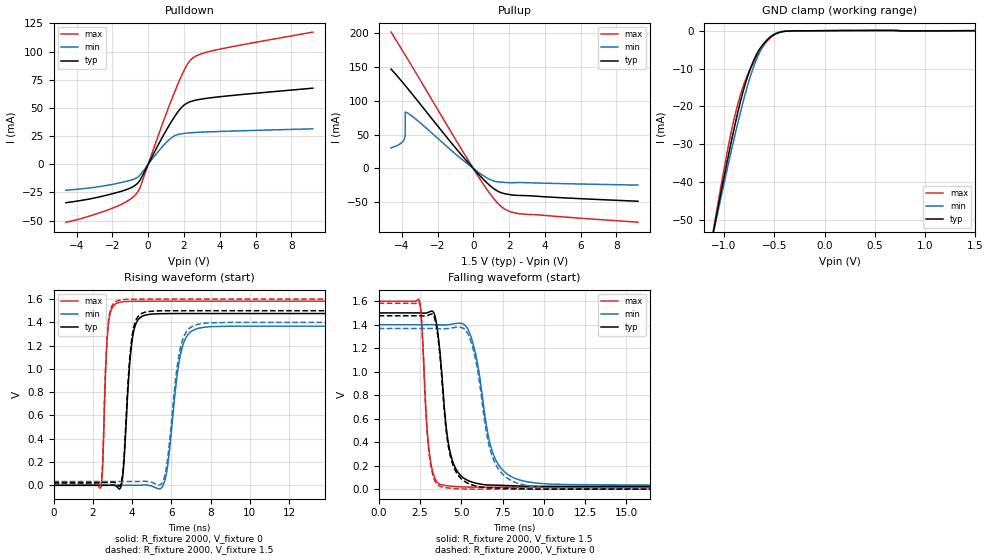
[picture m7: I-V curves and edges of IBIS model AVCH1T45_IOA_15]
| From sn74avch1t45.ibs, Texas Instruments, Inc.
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[Model]   AVCH1T45_IOA_15
Model_type  I/O
Vinl=0.49
Vinh=1.04
Enable   Active-Low
Vref =   0
Rref =   2000
Cref =   15p
Vmeas =   0.75
| variable   typ   min   max
C_comp   5.30pF   4.64pF   5.89pF
| C_pullup   5.23pF   3.72pF   7.65pF
| C_pulldown   4.92pF   4.34pF   5.58pF
| C_tri-state   5.30pF   4.64pF   5.89pF
[Temperature Range]   40   100   -40
| Ambient temperature   25   85   -40
[Voltage range]   1.5   1.4   1.6
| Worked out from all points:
|   slope of the pulldown table from 0 to 0.225 V, typ, clamps not added: 32.1 ohm
|   slope of the pullup table from 0 to 0.225 V, typ, clamps not added: 33.9 ohm
|   GND clamp passes 1 mA (typ) near -0.50 V on its own axis
|   rising waveform, R_fixture 2000, V_fixture 0: 20-80 % time 334ps typ, 544ps min, 203ps max; typ from 0 V to 1.48 V
|   falling waveform, R_fixture 2000, V_fixture 1.5: 20-80 % time 639ps typ, 1.02ns min, 391ps max; typ from 1.5 V to 0.023 V
|   rising waveform, R_fixture 2000, V_fixture 1.5: 20-80 % time 330ps typ, 532ps min, 202ps max; typ from 0.023 V to 1.5 V
|   falling waveform, R_fixture 2000, V_fixture 0: 20-80 % time 639ps typ, 1.01ns min, 386ps max; typ from 1.48 V to 0 V
[GND Clamp]
| AVCH1T45_IOA_15
|   Voltage   I(typ)   I(min)   I(max)
-4.6V     -599.6mA   -548.2mA   -664.6mA
-1.1V     -52.36mA   -52.8mA    -51.85mA
-1.075V   -48.9mA    -49.67mA   -47.95mA
-930mV    -29.68mA   -32.07mA   -27.01mA
-880mV    -23.6mA    -26.34mA   -21.2mA
-830mV    -18.08mA   -20.9mA    -16.41mA
-765mV    -12.13mA   -14.48mA   -11.64mA
-685mV    -6.738mA   -8.147mA   -7.41mA
-605mV    -3.434mA   -3.729mA   -3.946mA
-535mV    -1.679mA   -1.475mA   -1.741mA
-370mV    -121.9uA   -99.54uA   -128.4uA
1.5V      812pA      11.73uA    -26.87uA
[Pulldown]
| AVCH1T45_IOA_15
|   Voltage   I(typ)   I(min)   I(max)
-4.6V     -34.07mA   -23.01mA   -51.35mA
-1.88V    -25.6mA    -17.43mA   -38.2mA
-1.09V    -21.68mA   -14.59mA   -31.97mA
-630mV    -17.39mA   -11.88mA   -25.55mA
-415mV    -12.94mA   -8.777mA   -18.95mA
595mV     18.22mA    11.97mA    26.91mA
1.27V     37.14mA    23.08mA    55.77mA
1.7V      47.29mA    26.56mA    72.61mA
2.03V     52.78mA    27.45mA    84.03mA
2.5V      56.24mA    28.09mA    94.31mA
3.84V     59.63mA    29.04mA    101.6mA
9.2V      67.51mA    31.46mA    117.2mA
[Pullup]
| AVCH1T45_IOA_15
|   Voltage   I(typ)   I(min)   I(max)
-4.6V     146.8mA    30.47mA    201.5mA
-4.1V     131.8mA    36.24mA    180.2mA
-3.85V    123.9mA    43.97mA    169.4mA
-3.81V    122.6mA    49.37mA    167.6mA
-3.805V   122.5mA    83.3mA     167.4mA
-3.785V   121.8mA    83.17mA    166.5mA
-3.155V   101.3mA    71.56mA    138.9mA
175mV     -5.197mA   -3.574mA   -7.497mA
980mV     -26.35mA   -16.94mA   -39.04mA
1.625V    -36.35mA   -20.39mA   -57.65mA
2.595V    -39.89mA   -20.78mA   -66.9mA
9.2V      -48.41mA   -24.54mA   -79.36mA
[Ramp]
| AVCH1T45_IOA_15
| variable   typ   min   max
dV/dt_r   0.91/3.44E-10   0.84/5.58E-10   0.96/2.08E-10
dV/dt_f   0.90/6.47E-10   0.83/1.02E-09   0.96/3.96E-10
R_load = 2000
[Rising Waveform]
| AVCH1T45_IOA_15
R_fixture =   2000
C_fixture =   0
L_fixture =   0
V_fixture =   0
V_fixture_min = 0
V_fixture_max = 0
|   Time   V(typ)   V(min)   V(max)
0s        19.41nV    97.7nV     527.2pV
2.425ns   23.65uV    1.708uV    -13.22mV
2.78ns    -69.1uV    -12.18uV   1.359V
3.33ns    -29.77mV   11.82uV    1.571V
4.015ns   1.261V     -139.9uV   1.581V
4.68ns    1.463V     2.673mV    1.582V
5.64ns    1.475V     25.12mV    1.582V
6.48ns    1.476V     1.136V     1.582V
7.37ns    1.476V     1.349V     1.582V
34.99ns   1.476V     1.367V     1.582V
[Falling Waveform]
| AVCH1T45_IOA_15
R_fixture =   2000
C_fixture =   0
L_fixture =   0
V_fixture =   1.5
V_fixture_min = 1.4
V_fixture_max = 1.6
|   Time   V(typ)   V(min)   V(max)
0s        1.5V       1.4V       1.6V
2.46ns    1.5V       1.4V       1.607V
3.06ns    1.508V     1.4V       322mV
3.765ns   1.083V     1.398V     39.26mV
4.185ns   423.8mV    1.399V     28.99mV
4.745ns   155.9mV    1.411V     21.19mV
5.705ns   58.29mV    1.245V     17.52mV
6.975ns   34.14mV    285mV      17.14mV
8.5ns     27.07mV    79.24mV    17.11mV
34.99ns   23.4mV     32.34mV    17.1mV
[Rising Waveform]
| AVCH1T45_IOA_15
R_fixture =   2000
C_fixture =   0
L_fixture =   0
V_fixture =   1.5
V_fixture_min = 1.4
V_fixture_max = 1.6
|   Time   V(typ)   V(min)   V(max)
0s        23.4mV     32.34mV    17.1mV
2.425ns   23.42mV    32.34mV    4.596mV
2.775ns   23.31mV    32.32mV    1.376V
3.315ns   -3.39mV    32.35mV    1.589V
4.005ns   1.286V     32.2mV     1.599V
4.64ns    1.486V     34.87mV    1.6V
5.62ns    1.499V     55.33mV    1.6V
6.44ns    1.5V       1.165V     1.6V
7.32ns    1.5V       1.382V     1.6V
34.99ns   1.5V       1.4V       1.6V
[Falling Waveform]
| AVCH1T45_IOA_15
R_fixture =   2000
C_fixture =   0
L_fixture =   0
V_fixture =   0
V_fixture_min = 0
V_fixture_max = 0
|   Time   V(typ)   V(min)   V(max)
0s        1.476V     1.367V     1.582V
2.46ns    1.476V     1.367V     1.588V
3.035ns   1.482V     1.367V     327mV
3.735ns   1.099V     1.366V     22.93mV
4.17ns    409.2mV    1.367V     11.23mV
4.73ns    136mV      1.378V     3.649mV
5.685ns   34.98mV    1.213V     371.7uV
6.93ns    10.72mV    259.6mV    38.49uV
8.49ns    3.323mV    46.84mV    7.839uV
34.99ns   65.47nV    1.654uV    57.62nV
